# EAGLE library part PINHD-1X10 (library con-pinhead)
PIN HEADER
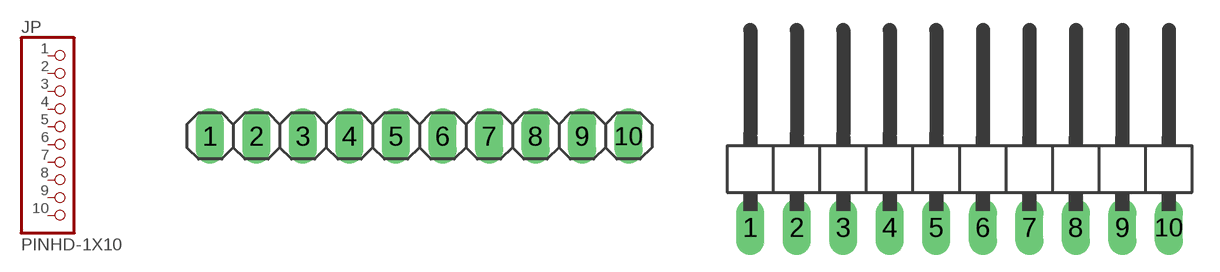
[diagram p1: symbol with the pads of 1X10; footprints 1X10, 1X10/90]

Designator prefix JP

## PINHD-1X10_2.54  [1X10]
1  1  pas
2  2  pas
3  3  pas
4  4  pas
5  5  pas
6  6  pas
7  7  pas
8  8  pas
9  9  pas
10  10  pas

## PINHD-1X10_2.54-90°  [1X10/90]
Pads as for 1X10

## PINHD-1X10_2.00  [1X10M]
Pads as for 1X10

## PINHD-1X10_2.54-SMD  [1X10SMD]
Pads as for 1X10

## PINHD-1X10_2.54-SMD-90°  [1X10SMD/90]
Pads as for 1X10

## Footprint 1X10 (pad centres in mm)
PIN HEADER - 2.54
drill 1.016 long: 1 -11.43,0; 2 -8.89,0; 3 -6.35,0; 4 -3.81,0; 5 -1.27,0; 6 1.27,0; 7 3.81,0; 8 6.35,0; 9 8.89,0; 10 11.43,0

## Footprint 1X10/90 (pad centres in mm)
PIN HEADER - 2.54 90°
drill 1.016 long: 1 -11.43,-3.81; 2 -8.89,-3.81; 3 -6.35,-3.81; 4 -3.81,-3.81; 5 -1.27,-3.81; 6 1.27,-3.81; 7 3.81,-3.81; 8 6.35,-3.81; 9 8.89,-3.81; 10 11.43,-3.81

## Footprint 1X10M (pad centres in mm)
PIN HEADER - 2
drill 0.914 square: 1 -9,0
drill 0.914: 2 -7,0; 3 -5,0; 4 -3,0; 5 -1,0; 6 1,0; 7 3,0; 8 5,0; 9 7,0; 10 9,0

## Footprint 1X10SMD (pad centres in mm)
PIN HEADER - 2.54 SMD
smd 1.016 x 3.302: 1 -1.27,1.27; 2 1.27,-1.27; 3 3.81,1.27; 4 6.35,-1.27; 5 8.89,1.27; 6 11.43,-1.27; 7 13.97,1.27; 8 16.51,-1.27; 9 19.05,1.27; 10 21.59,-1.27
